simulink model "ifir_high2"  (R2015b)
settings: Solver=VariableStepAuto  StartTime=0.0  StopTime=1  RelTol=1e-3
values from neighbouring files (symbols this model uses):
  delay = 2*nord1/2 + (nord2/2)*M1-1    (= 1535)    [basisband_2.m]    (also in ifir_dezim_1.m = fix((length(himage)-1)/2 + 5*(length(h)-1)/2); ifir_high_2.m = length(d)-1; ifir_interp_1.m = fix((length(h)-1)/2 + (length(himage)-1)/(2*L)))
  fg1 = 200    [ifir_high_2.m]
  fg2 = ',     num2str(fg2),' Hz (Ausgang des Blocks Delay)'])    [ifir_high_2.m]
  hup = -hup    [ifir_high1.m]    (also in ifir_high_2.m)
  L = 3    [farrow_3.m]    (also in farrow_4.m = 480; ifir_1.m = 5; ifir_dezim_1.m = 5; ifir_high1.m = 5)
  Ts = 1/fs    (= 5e-05)    [basisband_1.m]    (also in basisband_2.m = 5e-06; dezimier_1.m = 0.0005; dezimier_11.m = 0.0005; dezimier_2.m = 0.0005)
undefined symbols (not defined in the file or in its folder): hsupp

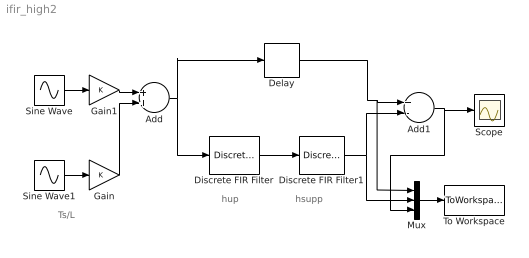
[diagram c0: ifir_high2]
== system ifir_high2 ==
  note: Ts/L
  note: hsupp
  note: hup
  Add : Sum
  Add1 : Sum  Inputs=+-
  Delay : Delay  DelayLength=delay
  Discrete FIR Filter : DiscreteFir  Coefficients=hup
  Discrete FIR Filter1 : DiscreteFir  Coefficients=hsupp
  Gain : Gain
  Gain1 : Gain
  Mux : Mux  Inputs=3
  Scope : Scope
  Sine Wave : Sin  Frequency=2*pi*fg1  SampleTime=Ts/L
  Sine Wave1 : Sin  Frequency=2*pi*fg2  SampleTime=Ts/L
  To Workspace : ToWorkspace  VariableName=y  SaveFormat=Timeseries  SampleTime=-1
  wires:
  Sine Wave/1 -> Gain1/1
  Sine Wave1/1 -> Gain/1
  Add/1 -> Discrete FIR Filter/1, Delay/1
  Discrete FIR Filter/1 -> Discrete FIR Filter1/1
  Delay/1 -> Add1/1, Mux/1
  Discrete FIR Filter1/1 -> Mux/2, Add1/2
  Add1/1 -> Mux/3, Scope/1
  Gain/1 -> Add/2
  Gain1/1 -> Add/1
  Mux/1 -> To Workspace/1
